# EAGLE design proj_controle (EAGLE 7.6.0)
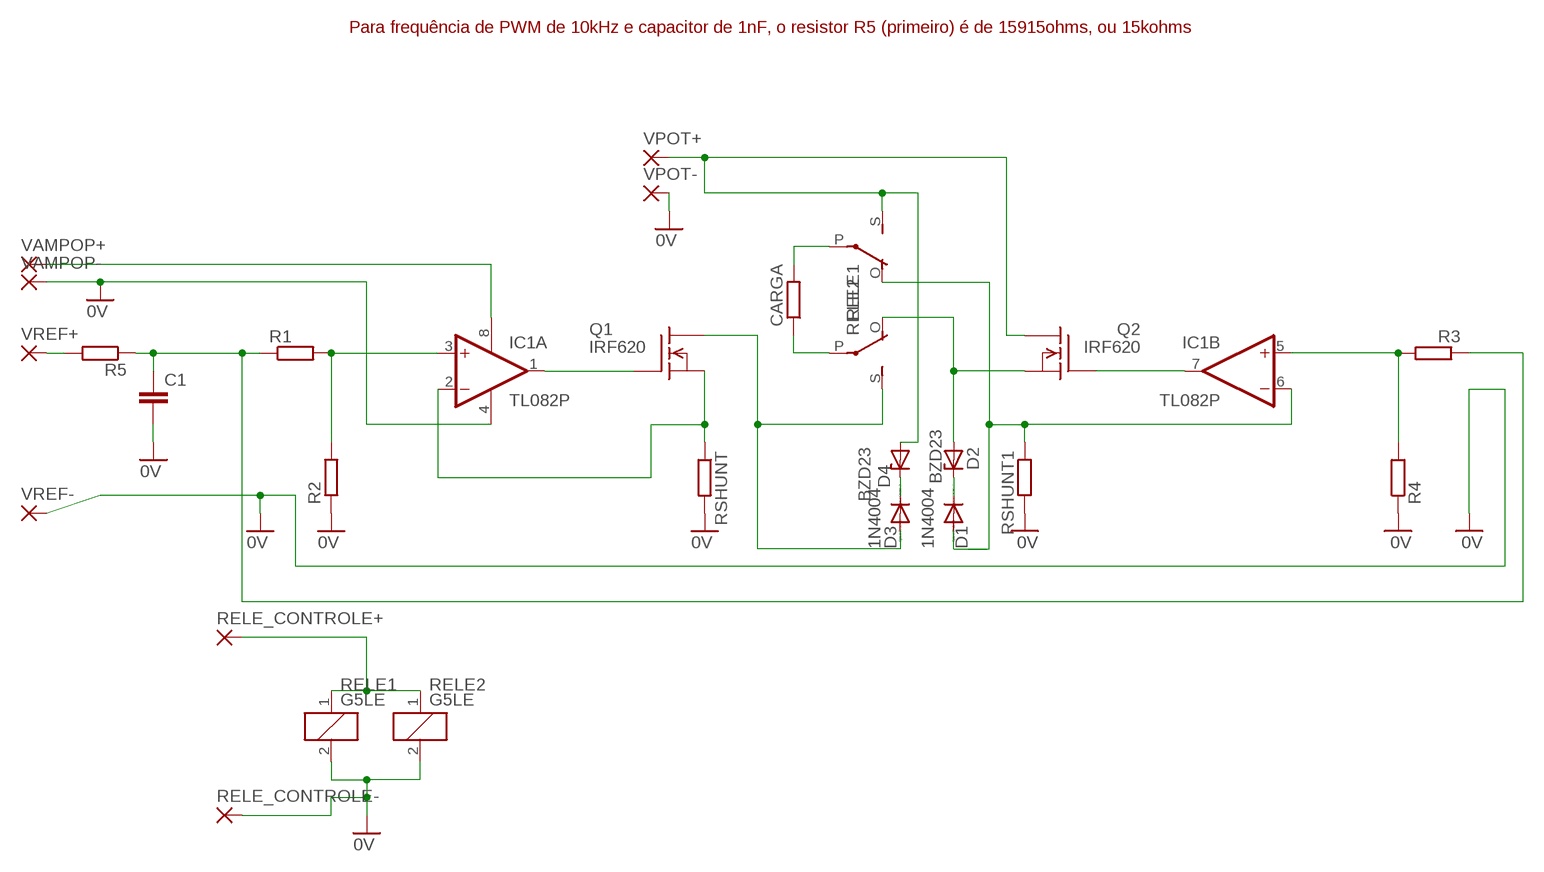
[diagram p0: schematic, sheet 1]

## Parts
C1  C-EU050-025X075  [C050-025X075]
CARGA  R-EU_0207/10  [0207/10]
D1  1N4004  [DO41-10]
D2  BZD23  [SOD81]
D3  1N4004  [DO41-10]
D4  BZD23  [SOD81]
IC1  TL082P  [DIL08]
Q1  IRF620  [TO220]
Q2  IRF620  [TO220]
R1  R-EU_0207/10  [0207/10]
R2  R-EU_0207/10  [0207/10]
R3  R-EU_0207/10  [0207/10]
R4  R-EU_0207/10  [0207/10]
R5  R-EU_0207/10  [0207/10]
RELE1  G5LE  [G5LE]
RELE2  G5LE  [G5LE]
RELE_CONTROLE+  3,17/1,1  [3,17/1,1]
RELE_CONTROLE-  3,17/1,1  [3,17/1,1]
RSHUNT  R-EU_0617/22  [0617/22]
RSHUNT1  R-EU_0617/22  [0617/22]
VAMPOP+  3,17/1,1  [3,17/1,1]
VAMPOP-  3,17/1,1  [3,17/1,1]
VPOT+  3,17/1,1  [3,17/1,1]
VPOT-  3,17/1,1  [3,17/1,1]
VREF+  3,17/1,1  [3,17/1,1]
VREF-  3,17/1,1  [3,17/1,1]

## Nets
0V: C1.2 IC1.4(P:V-) R2.1 R4.1 RELE1.2 RELE2.2 RELE_CONTROLE-.1(P) RSHUNT1.2 RSHUNT.2 VAMPOP-.1(P) VPOT-.1(P) VREF-.1(P)
N$1: CARGA.1 RELE2.P(2:P)
N$2: IC1.3(A:+IN) R1.2 R2.2
N$3: IC1.1(A:OUT) Q1.1(G)
N$5: C1.1 R1.1 R3.1 R5.1
N$6: R5.2 VREF+.1(P)
N$7: CARGA.2 RELE1.P(2:P)
N$8: D3.A Q1.2(D) RELE2.S(2:S)
N$9: IC1.5(B:+IN) R3.2 R4.2
N$10: IC1.7(B:OUT) Q2.1(G)
N$11: D1.A IC1.6(B:-IN) RELE1.O(2:O) RSHUNT1.1
N$12: D1.C D2.C
N$13: D4.A Q2.2(D) RELE1.S(2:S) VPOT+.1(P)
N$14: D2.A Q2.3(S) RELE2.O(2:O)
N$15: RELE1.1 RELE2.1 RELE_CONTROLE+.1(P)
N$16: D3.C D4.C
N$17: IC1.2(A:-IN) Q1.3(S) RSHUNT.1
N$18: IC1.8(P:V+) VAMPOP+.1(P)

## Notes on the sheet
- Para frequência de PWM de 10kHz e capacitor de 1nF, o resistor R5 (primeiro) é de 15915ohms, ou 15kohms

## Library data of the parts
C1 = rcl:C-EU: CAPACITOR, European symbol
CARGA R1-R5 = rcl:R-EU_: RESISTOR, European symbol
D1 D3 = diode:1N4004: DIODE
D2 D4 = diode:BZD23: Z DIODE
IC1 = linear:TL082: OP AMP Data sheet; DATA_SHEET: <a href="http://www.ti.com/lit/ds/symlink/tl084a.pdf"> Data sheet </a>
Q1 Q2 = transistor-fet:IRF620: N-Channel Enhancement MOSFET (HEXFET); 200V; 5,2A; 0,8Ohm
RELE1 RELE2 = relay:G5LE: RELAY 1 x switch, 10 A/120 V AC, 8 A/30 V DC, Omron; OC_FARNELL: unknown; OC_NEWARK: unknown
RELE_CONTROLE+ RELE_CONTROLE- VAMPOP+ VAMPOP- VPOT+ VPOT- VREF+ VREF- = wirepad:3,17/1,1: THROUGH-HOLE PAD
RSHUNT RSHUNT1 = resistor:R-EU_: RESISTOR, European symbol

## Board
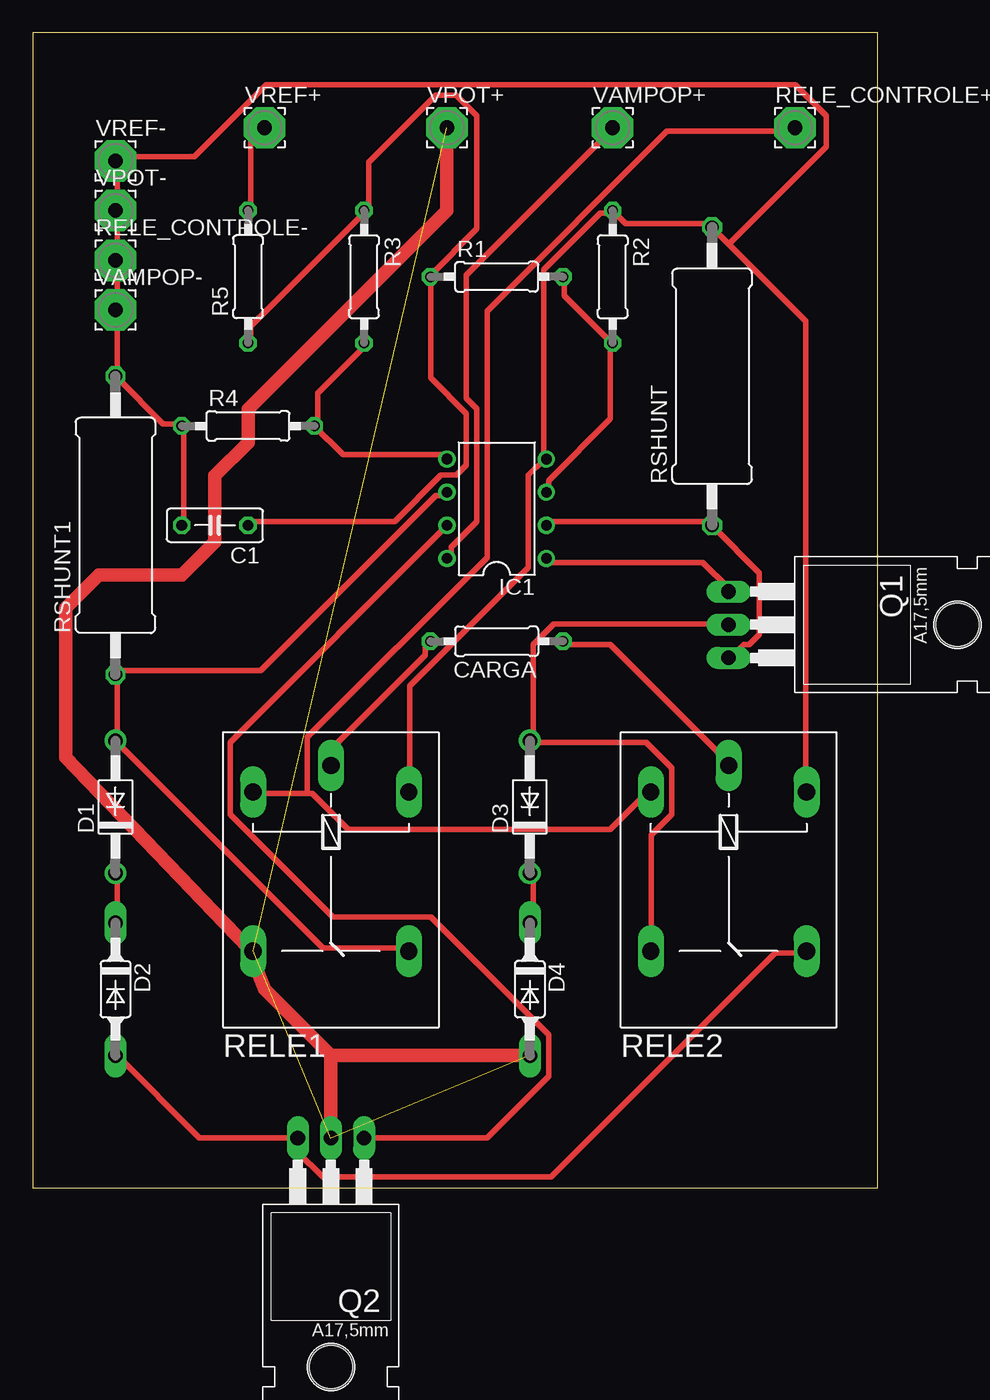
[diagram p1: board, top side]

Size 64.75 x 88.57 mm. Coordinates in mm from the lower left corner, seen from the top.
Outline: 0,0 64.75,0 64.75,88.57 0,88.57 0,0
Copper layers (1*16): Top 0.035mm / dielectric 1.5mm / Bottom 0.035mm
Design rules "default *": minimum track width 16mil, minimum drill 24mil, track to track 15mil, track to pad 15mil, pad to pad 15mil, via to via 15mil, smd to smd 8mil, copper to edge 40mil, drill to drill 8mil, minimum pad ring 10mil, minimum via ring 8mil, stop-mask expansion 4mil, vias tented up to drill 0mil, thermal gap 10mil

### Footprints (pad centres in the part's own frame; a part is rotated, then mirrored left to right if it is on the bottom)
C050-025X075 = drill 0.813 octagon: 1 -2.54,0; 2 2.54,0
0207/10 = drill 0.813 octagon: 1 -5.08,0; 2 5.08,0
DO41-10 = drill 1.118: A 5.08,0; C -5.08,0
SOD81 = drill 1.118 long: A 5.08,0; C -5.08,0
DIL08 = drill 0.813 pad 1.27: 1 -3.81,-3.81; 2 -1.27,-3.81; 3 1.27,-3.81; 4 3.81,-3.81; 5 3.81,3.81; 6 1.27,3.81; 7 -1.27,3.81; 8 -3.81,3.81
TO220 = drill 1.118 long: 1 -2.54,-6.35; 2 0,-6.35; 3 2.54,-6.35 | hole 3.302: 0,11.176
G5LE = drill 1.321 long: 1 -7.493,-5.969; 2 -7.493,5.969; O 4.699,5.969; P -9.525,0; S 4.699,-5.969
3,17/1,1 = drill 1.118 pad 3.175 octagon: 1 0,0
0617/22 = drill 1.016 octagon: 1 -11.43,0; 2 11.43,0

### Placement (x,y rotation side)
C1  13.97,50.8 180 top
CARGA  35.56,41.91 180 top
D1  6.35,29.21 90 top
D2  6.35,15.24 270 top
D3  38.1,29.21 90 top
D4  38.1,15.24 270 top
IC1  35.56,52.07 90 top
Q1  59.69,43.18 270 top
Q2  22.86,-2.54 180 top
R1  35.56,69.85 0 top
R2  44.45,69.85 270 top
R3  25.4,69.85 270 top
R4  16.51,58.42 0 top
R5  16.51,69.85 90 top
RELE1  22.86,22.86 270 top
RELE2  53.34,22.86 270 top
RELE_CONTROLE+  58.42,81.28 0 top
RELE_CONTROLE-  6.35,71.12 0 top
RSHUNT  52.07,62.23 90 top
RSHUNT1  6.35,50.8 90 top
VAMPOP+  44.45,81.28 0 top
VAMPOP-  6.35,67.31 0 top
VPOT+  31.75,81.28 0 top
VPOT-  6.35,74.93 0 top
VREF+  17.78,81.28 0 top
VREF-  6.35,78.74 0 top

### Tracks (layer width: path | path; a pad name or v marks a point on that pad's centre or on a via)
0V
  Top 0.406: C1.2 11.59,51.09 11.59,58.18 R4.1 11.2,58.57 10.02,58.57 6.48,62.12 RSHUNT1.2 6.48,62.51 6.48,67.23 VAMPOP-.1 6.48,67.63 6.48,70.78 RELE_CONTROLE-.1 6.48,71.17 6.48,74.71 VPOT-.1 6.48,75.11 6.48,78.65 VREF-.1 6.48,79.05 12.38,79.05 17.89,84.56 58.45,84.56 60.81,82.19 60.81,79.83 53.33,72.35 | RELE1.2 28.92,30.62 28.92,38.49 37.97,47.55 37.97,54.63 39.15,55.82 IC1.4 39.15,56.21 39.15,70.38 43.48,74.71 44.27,74.71 R2.1 45.45,73.93 51.75,73.93 RSHUNT.2 52.15,73.53 53.33,72.35 | 53.33,72.35 59.23,66.45 59.23,30.62 RELE2.2
N$1
  Top 0.406: CARGA.1 40.73,41.64 44.27,41.64 53.33,32.59 RELE2.P
N$2
  Top 0.406: IC1.3 39.55,53.45 39.55,54.24 44.27,58.97 44.27,64.48 R2.2 44.27,64.87 40.73,68.42 40.73,69.6 R1.2
N$3
  Top 0.406: IC1.1 39.55,47.94 51.36,47.94 53.33,45.97 Q1.1
N$5
  Top 0.406: R5.1 16.71,64.87 16.71,66.05 25.38,74.71 R3.1 25.77,75.11 25.77,78.65 30.89,83.77 32.46,83.77 34.04,82.19 34.04,73.53 30.49,69.99 R1.1 30.49,69.6 30.49,62.12 33.25,59.36 33.25,55.42 32.46,54.63 31.28,54.63 27.74,51.09 16.71,51.09 C1.1
N$6
  Top 0.406: R5.2 16.71,75.11 16.71,80.23 17.5,81.01 VREF+.1
N$7
  Top 0.406: CARGA.2 30.1,41.64 30.1,40.86 23.01,33.77 23.01,32.59 RELE1.P
N$8
  Top 0.406: Q1.2 53.33,43.22 39.94,43.22 38.37,41.64 38.37,34.56 D3.A 38.37,34.16 47.03,34.16 49,32.2 49,28.65 47.42,27.08 47.42,18.41 RELE2.S
N$9
  Top 0.406: R3.2 25.38,64.48 21.83,60.93 21.83,58.57 R4.2 23.8,56.21 31.67,56.21 IC1.5
N$10
  Top 0.406: IC1.7 31.67,50.7 15.14,34.16 15.14,28.65 23.01,20.78 30.49,20.78 39.55,11.72 39.55,8.57 34.82,3.85 25.77,3.85 Q2.1
N$11
  Top 0.406: IC1.6 31.67,53.06 30.89,53.06 17.5,39.67 6.48,39.67 RSHUNT1.1 6.48,39.28 6.48,34.56 D1.A 22.22,18.41 28.52,18.41 RELE1.O
N$12
  Top 0.406: D2.C 6.48,20.38 6.48,23.93 D1.C
N$13  (3 unrouted)
  Top 1.016: VPOT+.1 31.75,74.93 16.51,59.69 16.51,57.15 13.97,54.61 13.97,49.53 11.43,46.99 5.08,46.99 2.54,44.45 2.54,33.02 16.51,18.41 17.78,15.24 22.86,10.16 | 22.86,10.16 D4.A | Q2.2 22.86,10.16
N$14
  Top 0.406: D2.A 6.48,10.15 12.78,3.85 20.26,3.85 Q2.3 20.26,2.82 22.22,0.85 39.75,0.85 56.92,18.02 59.23,18.02 RELE2.O
N$15
  Top 0.406: 21.04,30.23 21.44,30.23 24.19,27.47 44.27,27.47 47.03,30.23 RELE2.1 | 21.04,30.23 17.11,30.23 RELE1.1 | 21.04,30.23 21.04,34.56 34.82,48.34 34.82,67.23 48.6,81.01 58.05,81.01 RELE_CONTROLE+.1
N$16
  Top 0.406: D4.C 38.37,20.38 38.37,23.93 D3.C
N$17
  Top 0.406: IC1.2 39.55,51.09 51.75,51.09 RSHUNT.1 52.15,50.7 55.69,47.15 55.69,42.43 54.9,41.64 54.51,41.64 53.72,40.86 Q1.3
N$18
  Top 0.406: IC1.8 32.07,48.34 32.07,49.12 34.04,51.09 34.04,59.75 33.25,60.54 33.25,69.99 44.27,81.01 VAMPOP+.1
